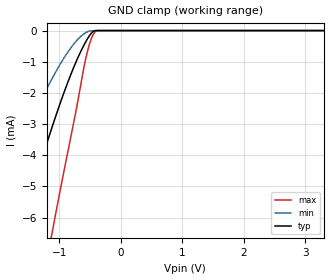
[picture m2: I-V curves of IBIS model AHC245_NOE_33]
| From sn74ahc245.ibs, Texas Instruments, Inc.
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[Model]   AHC245_NOE_33
Model_type  Input
Vinl = 0.9
Vinh = 2.1
| variable   typ   min   max
C_comp   0.74pF   0.66pF   0.81pF
[Temperature Range]   40   100   -40
| Ambient temperature   25   85   -40
[Voltage range]   3.3   3   3.6
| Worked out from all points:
|   GND clamp passes 1 mA (typ) near -0.73 V on its own axis
[GND Clamp]
| AHC245_NOE_33
|   Voltage   I(typ)   I(min)   I(max)
-3.3V     -19.16mA   -12.06mA   -33.37mA
-2.24V    -10.89mA   -6.576mA   -19.63mA
-2.19V    -10.51mA   -6.329mA   -19.01mA
-1.655V   -6.631mA   -3.784mA   -12.52mA
-1.605V   -6.284mA   -3.559mA   -11.93mA
-1.125V   -3.152mA   -1.574mA   -6.583mA
-1.085V   -2.913mA   -1.429mA   -6.164mA
-810mV    -1.404mA   -552.1uA   -3.398mA
-555mV    -312uA     -52.6uA    -780.8uA
-465mV    -59.32uA   -6.621uA   -198.1uA
-380mV    -31.36nA   -2.091uA   -157.8nA
3.3V      21.29pA    66.61pA    16.5pA
